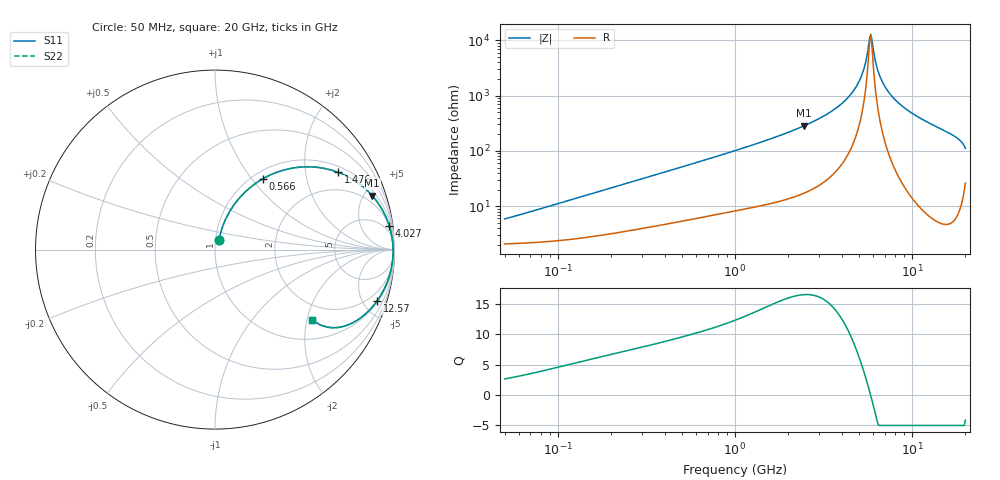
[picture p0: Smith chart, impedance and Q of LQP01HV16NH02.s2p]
!Murata Part Number: LQP01HV16NH02
!These Parameters are Measured in Series Mode Connection
!  o--[Z]--o
!Port1  Port2
!  o-------o
!Freq. Start=50[MHz] Stop=20[GHz], 401[Steps]
# Hz S RI R 50
!Freq.(Hz) S11(Real) S11(Imag) S21(Real) S21(Imag) S12(Real) S12(Imag) S22(Real) S22(Imag)
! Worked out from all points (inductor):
!   401 points, 50 MHz to 20 GHz, reference 50 ohm
!   read as one part in series: L = 17.4 nH near 58.08 MHz
!   highest Q = 16.5 at 2.456 GHz (marker M1), where L = 18.4 nH
!   self-resonance near 5.769 GHz
!   S11 on the Smith chart (normalised r, x): 50 MHz: 1.04, +0.11; 566 MHz: 1.12, +1.15; 1.476 GHz: 1.21, +3.03; 4.027 GHz: 2, +14; 12.57 GHz: 1.13, -6.30; 20 GHz: 1.52, -2.15
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5e7  0.0232 0.0525  0.9768 -0.0525  0.9768 -0.0525  0.0232 0.0525
1.364002e8  0.0453 0.1364  0.9547 -0.1364  0.9547 -0.1364  0.0453 0.1364
3.721004e8  0.156 0.3091  0.844 -0.3091  0.844 -0.3091  0.156 0.3091
5.659842e8  0.2688 0.3959  0.7312 -0.3959  0.7312 -0.3959  0.2688 0.3959
1e9  0.5038 0.4609  0.4962 -0.4609  0.4962 -0.4609  0.5038 0.4609
1.476162e9  0.686 0.4306  0.314 -0.4306  0.314 -0.4306  0.686 0.4306
2.456456e9  0.8754 0.3013  0.1246 -0.3013  0.1246 -0.3013  0.8754 0.3013
2.728004e9  0.903 0.2671  0.097 -0.2671  0.097 -0.2671  0.903 0.2671
4.026975e9  0.9711 0.132  0.0289 -0.132  0.0289 -0.132  0.9711 0.132
4.608136e9  0.9833 0.0841  0.0167 -0.0841  0.0167 -0.0841  0.9833 0.0841
5.041459e9  0.9886 0.0521  0.0114 -0.0521  0.0114 -0.0521  0.9886 0.0521
5.352748e9  0.9908 0.0307  0.0092 -0.0307  0.0092 -0.0307  0.9908 0.0307
5.683258e9  0.9921 0.00927  0.00793 -0.00927  0.00793 -0.00927  0.9921 0.00927
5.856089e9  0.9923 -0.00147  0.00767 0.00147  0.00767 0.00147  0.9923 -0.00147
5.944466e9  0.9924 -0.00685  0.00763 0.00685  0.00763 0.00685  0.9924 -0.00685
6.217679e9  0.9921 -0.023  0.00787 0.023  0.00787 0.023  0.9921 -0.023
6.503449e9  0.9913 -0.0392  0.00867 0.0392  0.00867 0.0392  0.9913 -0.0392
7.442007e9  0.9855 -0.0882  0.0145 0.0882  0.0145 0.0882  0.9855 -0.0882
9.178299e9  0.9654 -0.1657  0.0346 0.1657  0.0346 0.1657  0.9654 -0.1657
1.257102e10  0.9036 -0.285  0.0964 0.285  0.0964 0.285  0.9036 -0.285
1.721783e10  0.7712 -0.4058  0.2288 0.4058  0.2288 0.4058  0.7712 -0.4058
2e10  0.5414 -0.3917  0.4586 0.3917  0.4586 0.3917  0.5414 -0.3917
